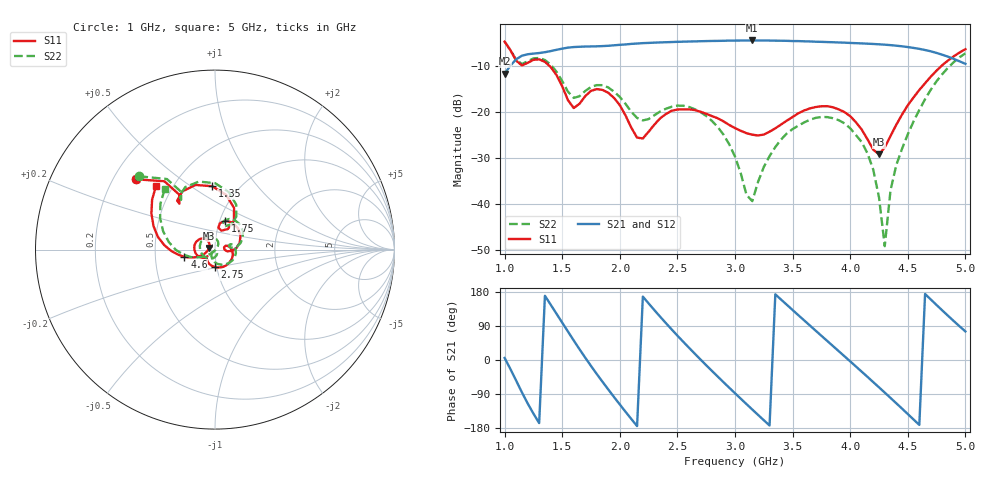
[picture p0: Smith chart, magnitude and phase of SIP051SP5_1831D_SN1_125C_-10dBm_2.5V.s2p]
# GHz  S  dB  R  50
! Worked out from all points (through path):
!   81 points, 1 GHz to 5 GHz, reference 50 ohm
!   highest |S21| = -4.38 dB at 3.15 GHz (marker M1); lowest = -11.6 dB at 1 GHz (marker M2)
!   lowest |S11| = -29.1 dB at 4.25 GHz (marker M3), VSWR 1.07, Z = 46.7 + j0.845 ohm
!   |S11| at or under -10 dB: 1.393 GHz to 4.789 GHz (3.396 GHz wide, 110 % of centre)
!   |S22| runs from -49.1 to -4.6 dB; largest |S21 - S12| = 0.0014
!   S11 on the Smith chart (normalised r, x): 1 GHz: 0.30, +0.35; 1.35 GHz: 0.76, +0.61; 1.75 GHz: 1.06, +0.35; 2.75 GHz: 0.98, -0.19; 4.6 GHz: 0.71, -0.06; 5 GHz: 0.40, +0.38
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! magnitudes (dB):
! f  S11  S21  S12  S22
! 1 GHz  -4.6  -11.6  -11.6  -4.6
! 1.15 GHz  -9.8  -7.7  -7.7  -9.5
! 1.35 GHz  -9.0  -6.9  -6.9  -8.6
! 1.6 GHz  -19.1  -5.8  -5.8  -16.9
! 1.7 GHz  -16.5  -5.7  -5.7  -15.4
! 1.75 GHz  -15.3  -5.7  -5.7  -14.5
! 1.95 GHz  -16.9  -5.4  -5.4  -15.5
! 2.15 GHz  -25.5  -5.0  -5.0  -21.2
! 2.35 GHz  -21.3  -4.8  -4.8  -19.8
! 2.75 GHz  -20.3  -4.5  -4.5  -20.8
! 3 GHz  -23.4  -4.4  -4.4  -29.6
! 3.15 GHz  -24.9  -4.4  -4.4  -39.3
! 3.35 GHz  -23.5  -4.4  -4.4  -27.5
! 3.7 GHz  -18.9  -4.7  -4.6  -21.2
! 3.9 GHz  -19.4  -4.8  -4.8  -21.7
! 4.1 GHz  -23.7  -5.0  -5.0  -26.5
! 4.25 GHz  -29.1  -5.2  -5.2  -38.5
! 4.3 GHz  -27.6  -5.3  -5.3  -49.1
! 4.35 GHz  -25.2  -5.4  -5.4  -37.0
! 4.45 GHz  -20.5  -5.7  -5.7  -27.9
! 4.6 GHz  -15.1  -6.2  -6.2  -19.5
! 5 GHz  -6.3  -9.5  -9.5  -7.2
